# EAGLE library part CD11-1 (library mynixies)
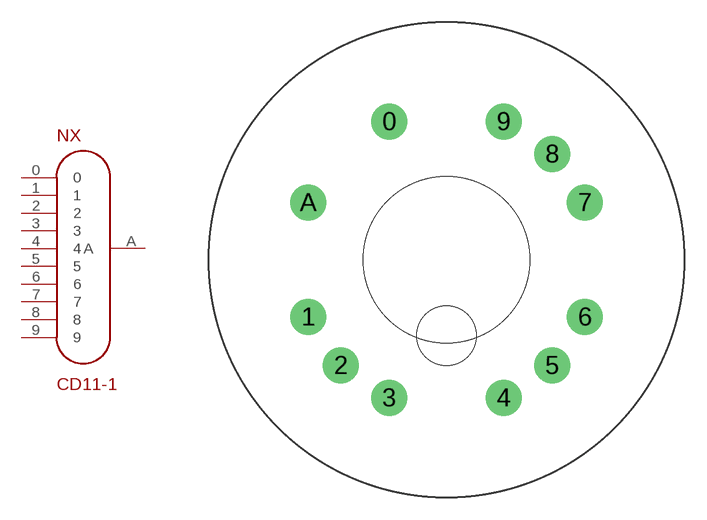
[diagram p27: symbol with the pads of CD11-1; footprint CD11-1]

Designator prefix NX

## CD11-1  [CD11-1]
0  0  pas
1  1  pas
2  2  pas
3  3  pas
4  4  pas
5  5  pas
6  6  pas
7  7  pas
8  8  pas
9  9  pas
A  A  pas

## Footprint CD11-1 (pad centres in mm)
drill 1.6: 0 -3.827,9.239; 1 -9.239,-3.827; 2 -7.071,-7.071; 3 -3.827,-9.239; 4 3.827,-9.239; 5 7.071,-7.071; 6 9.239,-3.827; 7 9.239,3.827; 8 7.071,7.071; 9 3.827,9.239; A -9.239,3.827
hole 11.113 at 0,0
hole 3.969 at 0,-5.08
